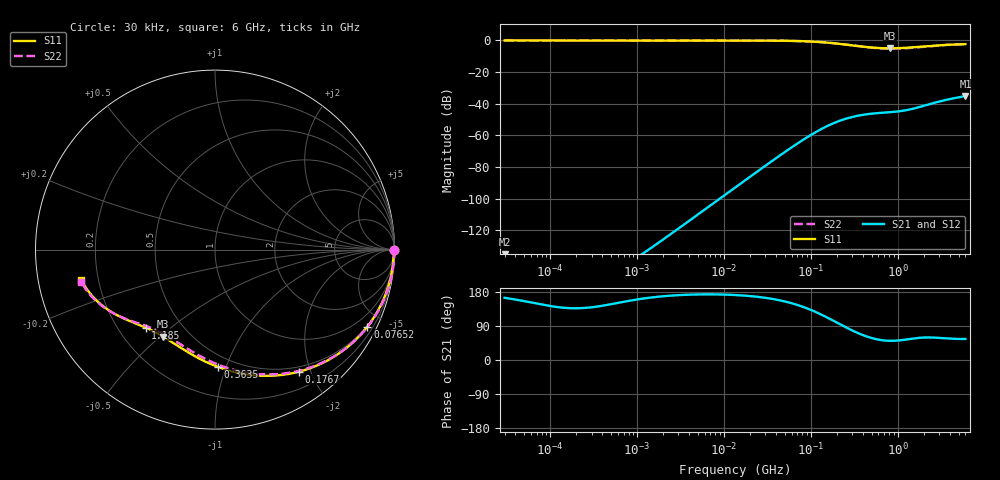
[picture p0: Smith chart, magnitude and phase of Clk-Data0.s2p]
!EMIF06-MSD04F3
!Simulation
!24/03/11  08:57
!Start Freq. :30.000kHz; Stop Freq. : 6.000GHz
!Number of points : 1592; Sweep : LOGARITHMIC
!B1-A1 (Clk-Data0)
!Freq ReS11 ImS11 ReS21 ImS21 ReS12 ImS12 ReS22 ImS22
# Hz  S  RI  R  50
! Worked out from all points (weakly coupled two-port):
!   1592 points, 30 kHz to 6 GHz, reference 50 ohm
!   highest |S21| = -35.14 dB at 6 GHz (marker M1); lowest = -184.8 dB at 30 kHz (marker M2)
!   lowest |S11| = -5.0 dB at 813.7 MHz (marker M3), VSWR 3.59, Z = 18 - j25.6 ohm
!   |S11| at or under -10 dB: nowhere
!   |S22| runs from -5.2 to 0.0 dB; largest |S21 - S12| = 3.4e-15
!   S11 on the Smith chart (normalised r, x): 30 kHz: open; 76.52 MHz: 0.46, -4.15; 176.7 MHz: 0.43, -1.83; 363.5 MHz: 0.41, -0.94; 1.185 GHz: 0.31, -0.41; 6 GHz: 0.14, -0.11
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30000  0.9996 -0.00136  -5.55e-10 1.58e-10  -5.55e-10 1.58e-10  1 -0.000184
231093.6  0.9967 -0.00267  -1.02e-08 9.5e-09  -1.02e-08 9.5e-09  1 -0.00142
1766531  0.9961 -0.0114  -3.95e-07 9.07e-08  -3.95e-07 9.07e-08  0.9999 -0.0108
5760426  0.9951 -0.0363  -4.13e-06 4.94e-07  -4.13e-06 4.94e-07  0.9991 -0.0353
1.350376e7  0.9909 -0.0845  -2.24e-05 3.36e-06  -2.24e-05 3.36e-06  0.9951 -0.0824
2.694354e7  0.9759 -0.1667  -8.64e-05 2.23e-05  -8.64e-05 2.23e-05  0.9806 -0.1626
2.864978e7  0.9733 -0.1769  -9.72e-05 2.65e-05  -9.72e-05 2.65e-05  0.9781 -0.1726
4.978761e7  0.9297 -0.2974  -0.000266 0.000126  -0.000266 0.000126  0.9362 -0.2904
7.652228e7  0.8495 -0.4288  -0.000515 0.000397  -0.000515 0.000397  0.8587 -0.4194
1.032257e8  0.7516 -0.5318  -0.00071 0.000818  -0.00071 0.000818  0.7638 -0.5212
1.340051e8  0.6306 -0.6156  -0.000788 0.00142  -0.000788 0.00142  0.6459 -0.6048
1.766531e8  0.4686 -0.6799  -0.000609 0.00225  -0.000609 0.00225  0.4871 -0.6702
2.495291e8  0.2423 -0.7021  0.000175 0.00332  0.000175 0.00332  0.2635 -0.6948
3.634583e8  0.0166 -0.6537  0.00152 0.004  0.00152 0.004  0.0389 -0.6489
5.213402e8  -0.1469 -0.5737  0.00268 0.00411  0.00268 0.00411  -0.1241 -0.57
7.890804e8  -0.2796 -0.4902  0.00341 0.00416  0.00341 0.00416  -0.2548 -0.4873
8.136818e8  -0.288 -0.4851  0.00344 0.00418  0.00344 0.00418  -0.263 -0.4824
1.18519e9  -0.3869 -0.4345  0.00364 0.00489  0.00364 0.00489  -0.3589 -0.4349
1.586553e9  -0.4652 -0.4023  0.0039 0.0061  0.0039 0.0061  -0.436 -0.4078
3.141386e9  -0.6435 -0.2987  0.00643 0.0103  0.00643 0.0103  -0.6256 -0.3168
4.403398e9  -0.7067 -0.2303  0.00834 0.0123  0.00834 0.0123  -0.699 -0.2478
6e9  -0.7453 -0.1673  0.00992 0.0144  0.00992 0.0144  -0.7453 -0.1796
